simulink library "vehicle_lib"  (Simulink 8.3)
settings: Solver=ode45  StartTime=0.0  StopTime=10.0  RelTol=1e-3
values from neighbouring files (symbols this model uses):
  ambient = class_REVS_ambient    [ambient_param.m]    (also in REVS_run_preproc.m)
  brake = struct(	'max_torque_Nm',[], 						'proportion_norm',1.0, 						'inertia_kgm2',0.0)    [class_REVS_drive_axle.m]
  driver = class_REVS_driver    [driver_param.m]    (also in REVS_run_preproc.m)
  final_drive = struct(	'gear_ratio',[], 								'efficiency_norm',[], 								'inertia_kgm2',[] )    [class_REVS_drive_axle.m]
  tire = struct(	'radius_m',[], 						'rolling_resistance_coefficient',0, 						'vehicle_weight_norm',1.0,  						'wheel_slip_torque_Nm',[],  						'inertia_kgm2',0.0)    [class_REVS_drive_axle.m]
  vehicle = class_REVS_vehicle    [vehicle_standard_car.m]
  vehicle_use_abc_roadload = true    [vehicle_standard_car.m]
undefined symbols (not defined in the file or in its folder): REVS, shaft
libraries: vehicle_lib x24, general_lib x13, audit_lib x12, simulink x7

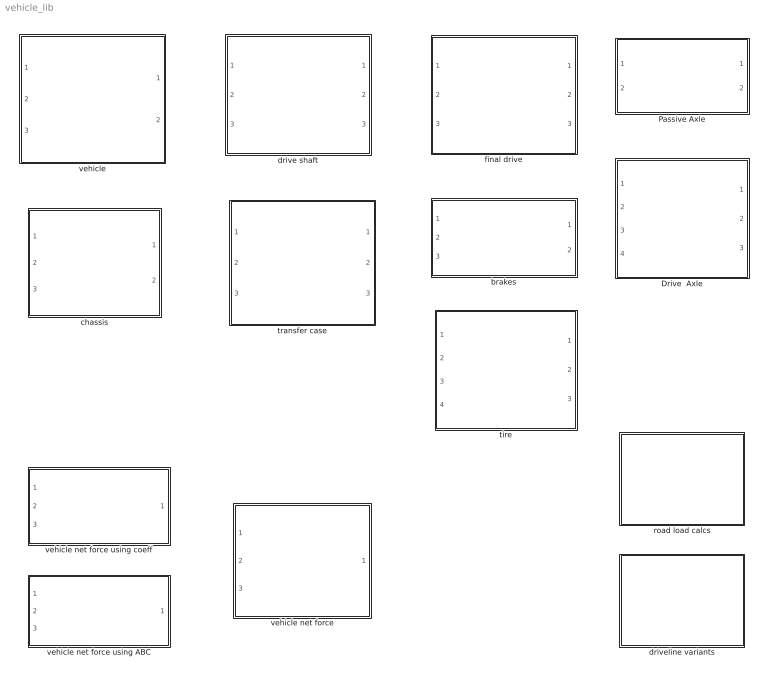
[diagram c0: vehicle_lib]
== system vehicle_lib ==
  Drive  Axle : Subsystem
  Passive Axle : Subsystem
  brakes : Subsystem
  chassis : Subsystem
  drive shaft : Subsystem
  driveline variants : Subsystem
  final drive : Subsystem
  road load calcs : Subsystem
  tire : Subsystem
  transfer case : Subsystem
  vehicle : Subsystem
  vehicle net force : Subsystem  Variant=on
  vehicle net force using ABC : Subsystem  VariantControl=vehicle_use_abc_roadload == true
  vehicle net force using coeff : Subsystem

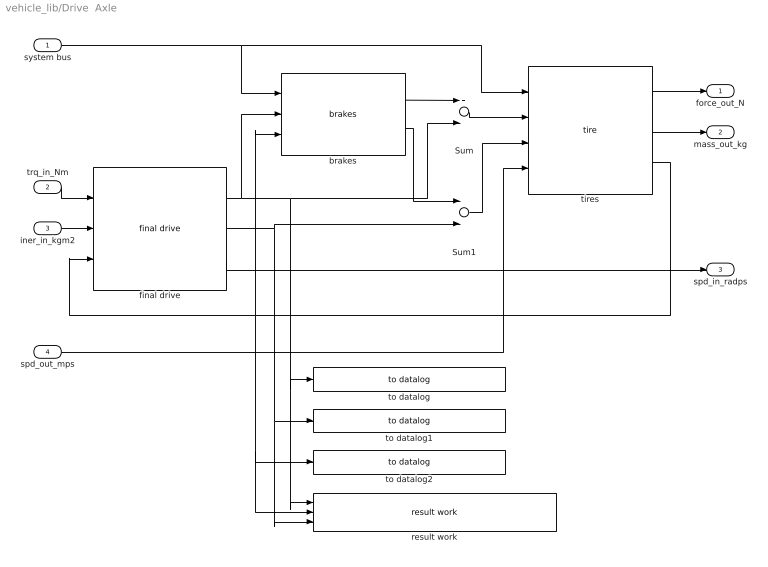
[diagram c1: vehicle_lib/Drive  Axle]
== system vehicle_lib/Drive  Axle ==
  system bus : Inport
  trq_in_Nm : Inport  Port=2
  iner_in_kgm2 : Inport  Port=3
  spd_out_mps : Inport  Port=4
  Sum : Sum
  Sum1 : Sum
  brakes : vehicle_lib/brakes  base_name=drive_axle1__brake  brake=axle.brake
  final drive : vehicle_lib/final drive  base_name=drive_axle1__final_drive  final_drive=axle.final_drive
  result work : general_lib/result work  ResultSignalName=axle_output_pos_work_kJ
  tires : vehicle_lib/tire  base_name=drive_axle1__tire  tire=axle.tire
  to datalog : general_lib/to datalog  VarName=final_drive.output_torque_Nm  WorkspaceName=datalog__final_drive__output_torque_Nm  VerboseLevel=0  VerboseSignal=REVS.verbose
  to datalog1 : general_lib/to datalog  VarName=final_drive.output_inertia_kgm2  WorkspaceName=datalog__final_drive__output_inertia_kgm2  VerboseLevel=0  VerboseSignal=REVS.verbose
  to datalog2 : general_lib/to datalog  VarName=final_drive.output_speed_radps  WorkspaceName=datalog__final_drive__output_speed_radps  VerboseLevel=0  VerboseSignal=REVS.verbose
  force_out_N : Outport
  mass_out_kg : Outport  Port=2
  spd_in_radps : Outport  Port=3
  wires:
  tires/2 -> mass_out_kg/1
  tires/1 -> force_out_N/1
  tires/3 -> result work/2, to datalog2/1, final drive/3, brakes/3
  spd_out_mps/1 -> tires/4
  system bus/1 -> tires/1, brakes/1
  Sum/1 -> tires/2
  brakes/1 -> Sum/1
  Sum1/1 -> tires/3
  brakes/2 -> Sum1/1
  trq_in_Nm/1 -> final drive/1
  iner_in_kgm2/1 -> final drive/2
  final drive/1 -> result work/1, to datalog/1, Sum/2, brakes/2
  final drive/2 -> result work/3, to datalog1/1, Sum1/2
  final drive/3 -> spd_in_radps/1

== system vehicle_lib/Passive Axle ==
  system bus : Inport
  spd_out_mps : Inport  Port=2
  Constant : Constant  Value=0
  brakes : vehicle_lib/brakes  base_name=steer_axle__brake  brake=axle.brake
  tires : vehicle_lib/tire  base_name=steer_axle__tire  tire=axle.tire
  force_out_N : Outport
  mass_out_kg : Outport  Port=2
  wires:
  brakes/1 -> tires/2
  system bus/1 -> tires/1, brakes/1
  brakes/2 -> tires/3
  spd_out_mps/1 -> tires/4
  tires/3 -> brakes/3
  tires/1 -> force_out_N/1
  tires/2 -> mass_out_kg/1
  Constant/1 -> brakes/2

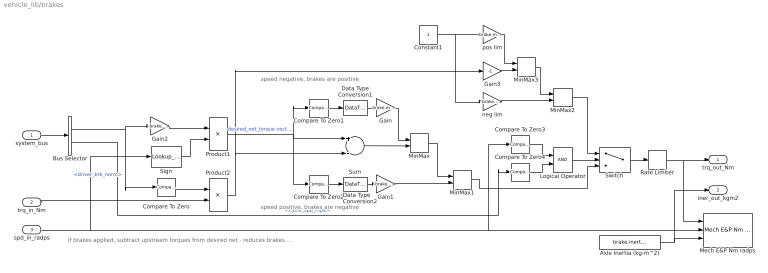
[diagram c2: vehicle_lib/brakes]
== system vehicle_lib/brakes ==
  note: speed negative, brakes are positive
  note: speed positive, brakes are negative
  note: if brakes applied, subtract upstream torques from desired net - reduces brakes for regen, increases if positive torques
  system_bus : Inport
  trq_in_Nm : Inport  Port=2
  spd_in_radps : Inport  Port=3
  Axle Inertia (kg-m^2) : Constant  Value=brake.inertia_kgm2
  Bus Selector : BusSelector  OutputSignals=driver.driver_brk_norm,driver.cycle_spd_mps
  Compare To Zero3 : simulink/Logic and Bit Operations/Compare To Zero  relop===  OutDataTypeStr=boolean
  Compare To Zero4 : simulink/Logic and Bit Operations/Compare To Zero  relop=<=  OutDataTypeStr=boolean
  Compare To Zero : simulink/Logic and Bit Operations/Compare To Zero  relop=>  OutDataTypeStr=boolean
  Compare To Zero1 : simulink/Logic and Bit Operations/Compare To Zero  relop=>  OutDataTypeStr=boolean
  Compare To Zero2 : simulink/Logic and Bit Operations/Compare To Zero  relop=<  OutDataTypeStr=boolean
  Constant1 : Constant
  Data Type Conversion1 : DataTypeConversion
  Data Type Conversion2 : DataTypeConversion
  Gain : Gain  Gain=brake.max_torque_Nm
  Gain1 : Gain  Gain=-brake.max_torque_Nm
  Gain2 : Gain  Gain=-brake.max_torque_Nm
  Gain3 : Gain  Gain=-1
  Logical Operator : Logic  AllPortsSameDT=off  OutDataTypeStr=boolean
  Mech E&P Nm radps : audit_lib/Mech E&P Nm radps  base_name=drive_axle1__brake  VerboseSignal=REVS.verbose
  MinMax : MinMax  Inputs=2  ZeroCross=off
  MinMax1 : MinMax  Function=max  Inputs=2  ZeroCross=off
  MinMax2 : MinMax  Function=max  Inputs=2  ZeroCross=off
  MinMax3 : MinMax  Inputs=2  ZeroCross=off
  Product1 : Product
  Product2 : Product
  Rate Limiter : RateLimiter  RisingSlewLimit=brake.max_torque_Nm  FallingSlewLimit=-brake.max_torque_Nm  SampleTimeMode=inherited
  Sign : Lookup_n-D  NumberOfTableDimensions=1  BreakpointsForDimension1=[-eps 0 eps]  BeginIndexSearchUsingPreviousIndexResult=on  Table=[-1 1 1]  ExtrapMethod=Clip  UseLastTableValue=on  RndMeth=Simplest
  Sum : Sum  Inputs=+-
  Switch : Switch  Criteria=u2 > Threshold
  neg lim : Gain  Gain=-brake.max_torque_Nm
  pos lim : Gain  Gain=brake.max_torque_Nm
  trq_out_Nm : Outport
  iner_out_kgm2 : Outport  Port=2
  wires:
  Constant1/1 -> pos lim/1, neg lim/1
  Switch/1 -> Rate Limiter/1
  MinMax2/1 -> Switch/1
  MinMax3/1 -> MinMax2/1
  neg lim/1 -> MinMax2/2
  Gain3/1 -> MinMax3/2
  pos lim/1 -> MinMax3/1
  MinMax1/1 -> Switch/3
  Logical Operator/1 -> Switch/2
  Product1/1 -> Compare To Zero2/1, Sum/1, Compare To Zero1/1  "desired_net_torque vector"
  Bus Selector/2 -> Compare To Zero4/1  "<cycle_spd_mps>"
  Compare To Zero4/1 -> Logical Operator/2
  Compare To Zero3/1 -> Logical Operator/1
  Rate Limiter/1 -> Mech E&P Nm radps/1, trq_out_Nm/1
  MinMax/1 -> MinMax1/1
  Gain2/1 -> Product1/1
  Sign/1 -> Product1/2
  system_bus/1 -> Bus Selector/1
  Axle Inertia (kg-m^2)/1 -> iner_out_kgm2/1, Mech E&P Nm radps/3
  spd_in_radps/1 -> Mech E&P Nm radps/2, Compare To Zero3/1, Sign/1
  Bus Selector/1 -> Compare To Zero/1, Gain2/1  "<driver_brk_norm>"
  trq_in_Nm/1 -> Product2/2
  Compare To Zero/1 -> Product2/1
  Product2/1 -> Sum/2, Gain3/1
  Sum/1 -> MinMax/2
  Compare To Zero1/1 -> Data Type Conversion1/1
  Gain/1 -> MinMax/1
  Compare To Zero2/1 -> Data Type Conversion2/1
  Gain1/1 -> MinMax1/2
  Data Type Conversion1/1 -> Gain/1
  Data Type Conversion2/1 -> Gain1/1

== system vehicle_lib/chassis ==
  system_bus : Inport
  force_in_N : Inport  Port=2
  mass_in_kg : Inport  Port=3
  Bus Creator : BusCreator  Inputs=2
  vehicle net force : vehicle_lib/vehicle net force
  vehicle speed integrator : Subsystem
  bus_out : Outport
  veh_spd_mps : Outport  Port=2
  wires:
  vehicle speed integrator/2(veh_dist_m) -> Bus Creator/2  "veh_dist_m"
  vehicle speed integrator/1(veh_spd_mps) -> veh_spd_mps/1, vehicle net force/3, Bus Creator/1  "veh_spd_mps"
  vehicle net force/1 -> vehicle speed integrator/1(force_out_N)
  mass_in_kg/1 -> vehicle speed integrator/2(mass_in_kg)
  force_in_N/1 -> vehicle net force/2
  system_bus/1 -> vehicle net force/1
  Bus Creator/1 -> bus_out/1  "vehicle"

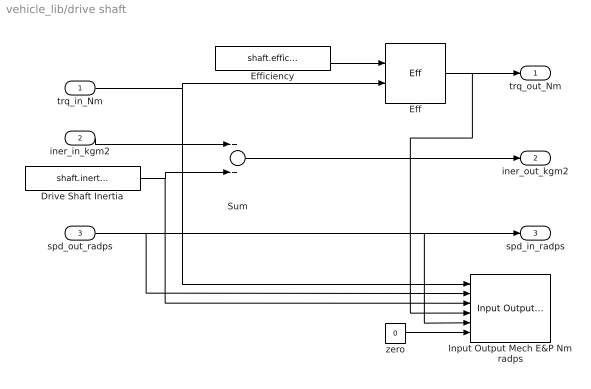
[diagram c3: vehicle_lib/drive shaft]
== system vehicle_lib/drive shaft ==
  trq_in_Nm : Inport
  iner_in_kgm2 : Inport  Port=2
  spd_out_radps : Inport  Port=3
  Drive Shaft Inertia : Constant  Value=shaft.inertia_kgm2
  Eff : general_lib/Eff
  Efficiency : Constant  Value=shaft.efficiency_norm
  Input Output Mech E&P Nm radps : audit_lib/Input Output Mech E&P Nm radps  base_name=driveshaft  VerboseSignal=REVS.verbose
  Sum : Sum
  zero : Constant  Value=0
  trq_out_Nm : Outport
  iner_out_kgm2 : Outport  Port=2
  spd_in_radps : Outport  Port=3
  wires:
  iner_in_kgm2/1 -> Sum/1
  Sum/1 -> iner_out_kgm2/1
  Drive Shaft Inertia/1 -> Input Output Mech E&P Nm radps/3, Sum/2
  spd_out_radps/1 -> Input Output Mech E&P Nm radps/2, Input Output Mech E&P Nm radps/5, spd_in_radps/1
  trq_in_Nm/1 -> Eff/2, Input Output Mech E&P Nm radps/1
  Efficiency/1 -> Eff/1
  Eff/1 -> Input Output Mech E&P Nm radps/4, trq_out_Nm/1
  zero/1 -> Input Output Mech E&P Nm radps/6

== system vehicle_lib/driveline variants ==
  driveline : Subsystem  Variant=on
  one axle drive : Subsystem  VariantControl=vehicle_driveline_type == enum_driveline_type.one_axle_drive

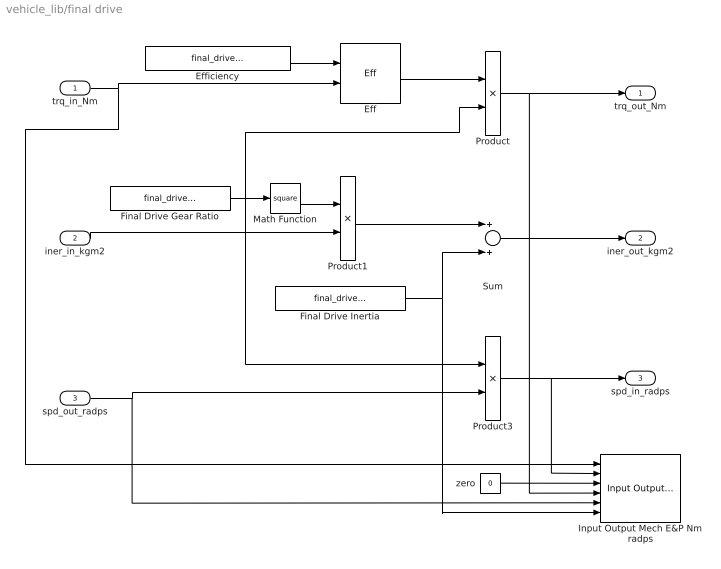
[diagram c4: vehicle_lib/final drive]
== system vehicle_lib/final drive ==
  trq_in_Nm : Inport
  iner_in_kgm2 : Inport  Port=2
  spd_out_radps : Inport  Port=3
  Eff : general_lib/Eff
  Efficiency : Constant  Value=final_drive.efficiency_norm
  Final Drive Gear Ratio : Constant  Value=final_drive.gear_ratio
  Final Drive Inertia : Constant  Value=final_drive.inertia_kgm2
  Input Output Mech E&P Nm radps : audit_lib/Input Output Mech E&P Nm radps  base_name=device  VerboseSignal=REVS.verbose
  Math Function : Math  Operator=square
  Product : Product
  Product1 : Product
  Product3 : Product
  Sum : Sum
  zero : Constant  Value=0
  trq_out_Nm : Outport
  iner_out_kgm2 : Outport  Port=2
  spd_in_radps : Outport  Port=3
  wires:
  Sum/1 -> iner_out_kgm2/1
  Product/1 -> Input Output Mech E&P Nm radps/4, trq_out_Nm/1
  Final Drive Inertia/1 -> Input Output Mech E&P Nm radps/6, Sum/2
  Product1/1 -> Sum/1
  iner_in_kgm2/1 -> Product1/2
  trq_in_Nm/1 -> Eff/2, Input Output Mech E&P Nm radps/1
  Final Drive Gear Ratio/1 -> Product/2, Math Function/1, Product3/1
  Math Function/1 -> Product1/1
  spd_out_radps/1 -> Input Output Mech E&P Nm radps/5, Product3/2
  Product3/1 -> Input Output Mech E&P Nm radps/2, spd_in_radps/1
  Efficiency/1 -> Eff/1
  Eff/1 -> Product/1
  zero/1 -> Input Output Mech E&P Nm radps/3

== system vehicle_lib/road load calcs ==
  acceleration force : Subsystem
  aerodynamic drag : Subsystem
  driver road load by ABC : Subsystem  InitFcn=if GEM_verbose disp('Using driver roadload by coastdown...'); end  VariantControl=variants_driver_roadload_ABC
  driver road load by Cd-Crr : Subsystem  InitFcn=if GEM_verbose disp('Using driver roadload by coefficients...'); end  VariantControl=variants_driver_roadload_coeff
  gradient force : Subsystem
  road load by ABC : Subsystem
  rolling resistance : Subsystem

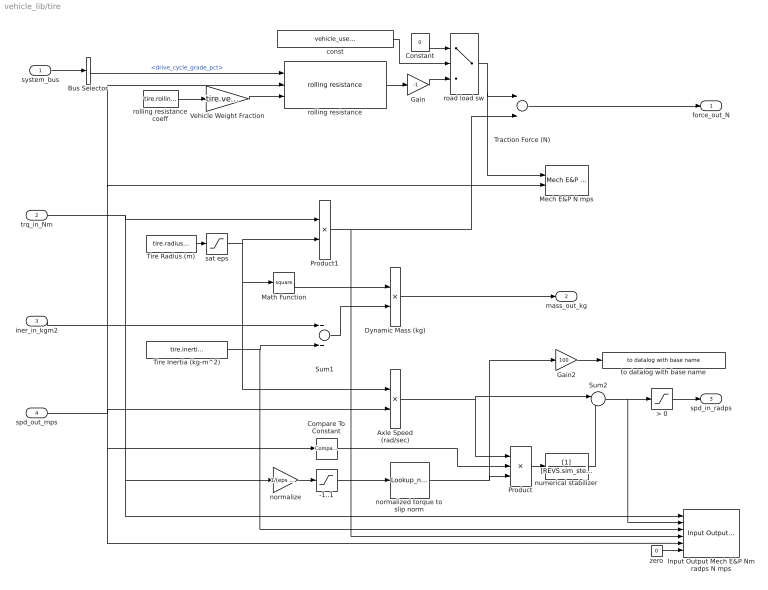
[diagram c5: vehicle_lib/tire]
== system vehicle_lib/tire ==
  system_bus : Inport
  trq_in_Nm : Inport  Port=2
  iner_in_kgm2 : Inport  Port=3
  spd_out_mps : Inport  Port=4
  -1..1 : Saturate  UpperLimit=1  LowerLimit=-1  ZeroCross=off
  > 0 : Saturate  UpperLimit=Inf  LowerLimit=0  ZeroCross=off
  Axle Speed (rad/sec) : Product  Inputs=/*
  Bus Selector : BusSelector  OutputSignals=ambient.drive_cycle_grade_pct
  Compare To Constant : simulink/Logic and Bit Operations/Compare To Constant  relop=>=  const=0.1  OutDataTypeStr=boolean
  Constant : Constant  Value=0
  Dynamic Mass (kg) : Product  Inputs=/*
  Gain : Gain  Gain=-1
  Gain2 : Gain  Gain=100
  Input Output Mech E&P Nm radps N mps : audit_lib/Input Output Mech E&P Nm radps N mps  base_name=drive_axle1__tire  VerboseSignal=REVS.verbose
  Math Function : Math  Operator=square
  Mech E&P N mps : audit_lib/Mech E&P N mps0  base_name=drive_axle1__tire__rolling_drag  VerboseSignal=REVS.verbose
  Product : Product  Inputs=3
  Product1 : Product  Inputs=*/
  Sum1 : Sum
  Sum2 : Sum  Inputs=|++
  Tire Inertia (kg-m^2) : Constant  Value=tire.inertia_kgm2
  Tire Radius (m) : Constant  Value=tire.radius_m
  Traction Force (N) : Sum
  Vehicle Weight Fraction : Gain  Gain=tire.vehicle_weight_norm
  const : Constant  Value=vehicle_use_abc_roadload
  normalize : Gain  Gain=1/(eps + tire.wheel_slip_torque_Nm)
  normalized torque to slip norm : Lookup_n-D  NumberOfTableDimensions=1  BreakpointsForDimension1=[-0.999866216844745 -0.99978414282011 -0.99807408909811 -0.994136683198638 -0.987125284420945 -0.975823606608682 -0.958455233159564 -0.932389621966496 -0.893705646328621 -0.836611821621369 -0.752906045607232 -0.632208437687154 -0.464747309940849 -0.248771439727253 0 0.248771439727253 0.464747309940849 0.632208437687154 0.752906045607232 0.836611821621369 0.893705646328621 0.932389621966496 0.95845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  IndexSearchMethod=Linear search  BeginIndexSearchUsingPreviousIndexResult=on  Table=-0.14 : 0.01 : 0.14  ExtrapMethod=Clip  UseLastTableValue=on  RndMeth=Simplest
  numerical stabilizer : TransferFcn  Denominator=[REVS.sim_step_time_secs 1]
  road load sw : Switch  Criteria=u2 > Threshold  ZeroCross=off
  rolling resistance : vehicle_lib/road load calcs/rolling resistance
  rolling resistance coeff : Constant  Value=tire.rolling_resistance_coefficient
  sat eps : Saturate  UpperLimit=Inf  LowerLimit=eps  ZeroCross=off
  to datalog with base name : general_lib/to datalog with base name  varName=slip_pct  baseName=base_name  VerboseLevel=1  VerboseSignal=REVS.verbose
  zero : Constant  Value=0
  force_out_N : Outport
  mass_out_kg : Outport  Port=2
  spd_in_radps : Outport  Port=3
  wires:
  normalized torque to slip norm/1 -> Product/3, Gain2/1
  -1..1/1 -> normalized torque to slip norm/1
  Compare To Constant/1 -> Product/2
  normalize/1 -> -1..1/1
  Gain2/1 -> to datalog with base name/1
  > 0/1 -> spd_in_radps/1
  spd_out_mps/1 -> Mech E&P N mps/2, rolling resistance/2, Axle Speed (rad/sec)/2, Input Output Mech E&P Nm radps N mps/5, Compare To Constant/1
  numerical stabilizer/1 -> Sum2/2
  Sum2/1 -> > 0/1, Input Output Mech E&P Nm radps N mps/2
  Product/1 -> numerical stabilizer/1
  Traction Force (N)/1 -> force_out_N/1
  trq_in_Nm/1 -> Product1/1, normalize/1, Input Output Mech E&P Nm radps N mps/1
  Axle Speed (rad/sec)/1 -> Product/1, Sum2/1
  Vehicle Weight Fraction/1 -> rolling resistance/3
  rolling resistance/1 -> Gain/1
  Bus Selector/1 -> rolling resistance/1  "<drive_cycle_grade_pct>"
  rolling resistance coeff/1 -> Vehicle Weight Fraction/1
  Dynamic Mass (kg)/1 -> mass_out_kg/1
  Sum1/1 -> Dynamic Mass (kg)/2
  Tire Inertia (kg-m^2)/1 -> Sum1/2, Input Output Mech E&P Nm radps N mps/3
  iner_in_kgm2/1 -> Sum1/1
  Tire Radius (m)/1 -> sat eps/1
  system_bus/1 -> Bus Selector/1
  Product1/1 -> Input Output Mech E&P Nm radps N mps/4, Traction Force (N)/2
  road load sw/1 -> Mech E&P N mps/1, Traction Force (N)/1
  Gain/1 -> road load sw/3
  const/1 -> road load sw/2
  Constant/1 -> road load sw/1
  sat eps/1 -> Axle Speed (rad/sec)/1, Math Function/1, Product1/2
  Math Function/1 -> Dynamic Mass (kg)/1
  zero/1 -> Input Output Mech E&P Nm radps N mps/6

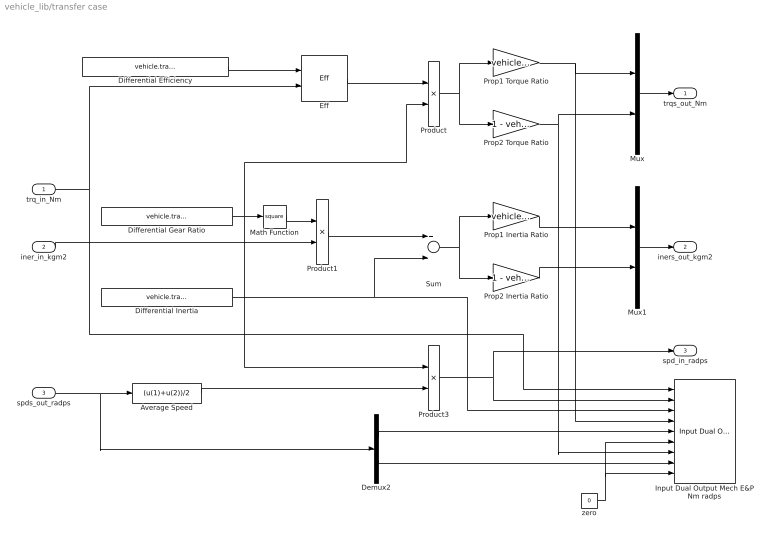
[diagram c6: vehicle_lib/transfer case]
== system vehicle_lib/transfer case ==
  trq_in_Nm : Inport
  iner_in_kgm2 : Inport  Port=2
  spds_out_radps : Inport  Port=3
  Average Speed : Fcn  Expr=(u(1)+u(2))/2
  Demux2 : Demux  Outputs=2
  Differential Efficiency : Constant  Value=vehicle.transfer_case.efficiency_norm
  Differential Gear Ratio : Constant  Value=vehicle.transfer_case.gear_ratio
  Differential Inertia : Constant  Value=vehicle.transfer_case.inertia_kgm2
  Eff : general_lib/Eff
  Input Dual Output Mech E&P Nm radps : audit_lib/Input Dual Output Mech E&P Nm radps  base_name=transfer_case  VerboseSignal=REVS.verbose
  Math Function : Math  Operator=square
  Mux : Mux  Inputs=2
  Mux1 : Mux  Inputs=2
  Product : Product
  Product1 : Product
  Product3 : Product
  Prop1 Inertia Ratio : Gain  Gain=vehicle.transfer_case.prop1_torque_ratio
  Prop1 Torque Ratio : Gain  Gain=vehicle.transfer_case.prop1_torque_ratio
  Prop2 Inertia Ratio : Gain  Gain=1 - vehicle.transfer_case.prop1_torque_ratio
  Prop2 Torque Ratio : Gain  Gain=1 - vehicle.transfer_case.prop1_torque_ratio
  Sum : Sum
  zero : Constant  Value=0
  trqs_out_Nm : Outport
  iners_out_kgm2 : Outport  Port=2
  spd_in_radps : Outport  Port=3
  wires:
  Demux2/2 -> Input Dual Output Mech E&P Nm radps/8
  Demux2/1 -> Input Dual Output Mech E&P Nm radps/5
  Average Speed/1 -> Product3/2
  spds_out_radps/1 -> Average Speed/1, Demux2/1
  Math Function/1 -> Product1/1
  Differential Gear Ratio/1 -> Math Function/1, Product/2, Product3/1
  trq_in_Nm/1 -> Eff/2, Input Dual Output Mech E&P Nm radps/1
  Eff/1 -> Product/1
  iner_in_kgm2/1 -> Product1/2
  Product1/1 -> Sum/1
  Differential Inertia/1 -> Sum/2, Input Dual Output Mech E&P Nm radps/3
  Product3/1 -> Input Dual Output Mech E&P Nm radps/2, spd_in_radps/1
  Product/1 -> Prop1 Torque Ratio/1, Prop2 Torque Ratio/1
  Sum/1 -> Prop1 Inertia Ratio/1, Prop2 Inertia Ratio/1
  Prop1 Torque Ratio/1 -> Input Dual Output Mech E&P Nm radps/4, Mux/1
  Prop2 Torque Ratio/1 -> Input Dual Output Mech E&P Nm radps/7, Mux/2
  Prop1 Inertia Ratio/1 -> Mux1/1
  Prop2 Inertia Ratio/1 -> Mux1/2
  Mux/1 -> trqs_out_Nm/1
  Mux1/1 -> iners_out_kgm2/1
  Differential Efficiency/1 -> Eff/1
  zero/1 -> Input Dual Output Mech E&P Nm radps/6, Input Dual Output Mech E&P Nm radps/9

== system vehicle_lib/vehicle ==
  system_bus : Inport
  trq_in_Nm : Inport  Port=2
  iner_in_kgm2 : Inport  Port=3
  Bus Creator1 : BusCreator  Inputs=1
  chassis : vehicle_lib/chassis  SystemSampleTime=-1
  driveline : vehicle_lib/driveline variants/driveline
  bus_out : Outport
  spd_in_radps : Outport  Port=2
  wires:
  chassis/2 -> driveline/4
  system_bus/1 -> driveline/1, chassis/1
  trq_in_Nm/1 -> driveline/2
  iner_in_kgm2/1 -> driveline/3
  driveline/3 -> spd_in_radps/1
  driveline/1 -> chassis/2
  driveline/2 -> chassis/3
  chassis/1 -> Bus Creator1/1  "chassis"
  Bus Creator1/1 -> bus_out/1  "vehicle"

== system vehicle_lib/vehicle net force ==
  note: 1) Only subsystems can be added as variant choices at this level 2) Blocks cannot be connected at this level as connectivity is automatically determined at simulation, based on the active variant
  system_bus : Inport
  force_in_N : Inport  Port=2
  chs_spd_mps : Inport  Port=3
  vehicle net force using ABC : vehicle_lib/vehicle net force using ABC  VariantControl=vehicle_use_abc_roadload == true
  vehicle net force using coeff : vehicle_lib/vehicle net force using coeff  VariantControl=vehicle_use_abc_roadload == false
  force_out_N : Outport

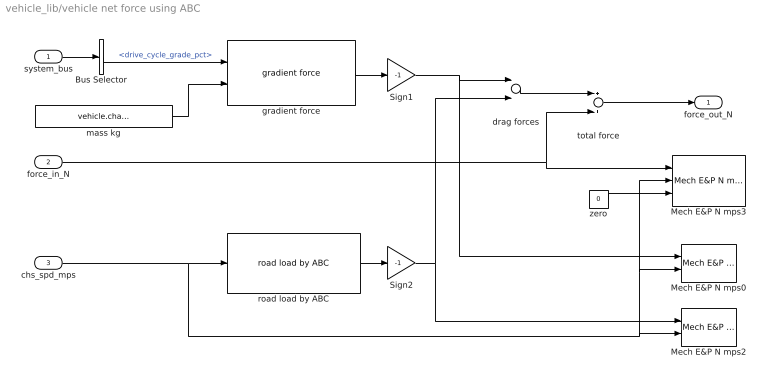
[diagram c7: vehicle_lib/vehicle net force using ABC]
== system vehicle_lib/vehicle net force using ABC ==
  system_bus : Inport
  force_in_N : Inport  Port=2
  chs_spd_mps : Inport  Port=3
  Bus Selector : BusSelector  OutputSignals=ambient.drive_cycle_grade_pct
  Mech E&P N mps0 : audit_lib/Mech E&P N mps0  base_name=vehicle.gradient_drag  VerboseSignal=REVS.verbose
  Mech E&P N mps2 : audit_lib/Mech E&P N mps0  base_name=vehicle.ABC_drag  VerboseSignal=REVS.verbose
  Mech E&P N mps3 : audit_lib/Mech E&P N mps  base_name=vehicle.input  VerboseSignal=REVS.verbose
  Sign1 : Gain  Gain=-1
  Sign2 : Gain  Gain=-1
  drag forces : Sum
  gradient force : vehicle_lib/road load calcs/gradient force
  mass kg : Constant  Value=vehicle.chassis.mass_static_kg
  road load by ABC : vehicle_lib/road load calcs/road load by ABC
  total force : Sum
  zero : Constant  Value=0
  force_out_N : Outport
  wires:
  zero/1 -> Mech E&P N mps3/3
  chs_spd_mps/1 -> road load by ABC/1, Mech E&P N mps2/2, Mech E&P N mps0/2, Mech E&P N mps3/2
  gradient force/1 -> Sign1/1
  drag forces/1 -> total force/1
  Sign1/1 -> Mech E&P N mps0/1, drag forces/1
  Bus Selector/1 -> gradient force/1  "<drive_cycle_grade_pct>"
  system_bus/1 -> Bus Selector/1
  mass kg/1 -> gradient force/2
  force_in_N/1 -> total force/2, Mech E&P N mps3/1
  total force/1 -> force_out_N/1
  road load by ABC/1 -> Sign2/1
  Sign2/1 -> drag forces/2, Mech E&P N mps2/1

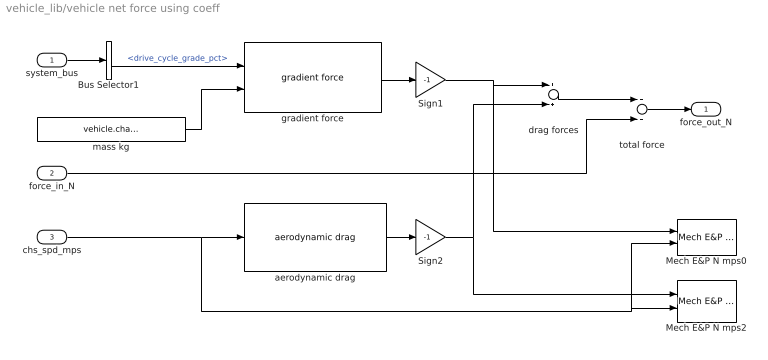
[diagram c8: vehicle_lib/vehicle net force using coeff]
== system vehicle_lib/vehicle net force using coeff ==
  system_bus : Inport
  force_in_N : Inport  Port=2
  chs_spd_mps : Inport  Port=3
  Bus Selector1 : BusSelector  OutputSignals=ambient.drive_cycle_grade_pct
  Mech E&P N mps0 : audit_lib/Mech E&P N mps0  base_name=vehicle.gradient_drag  VerboseSignal=REVS.verbose
  Mech E&P N mps2 : audit_lib/Mech E&P N mps0  base_name=vehicle.aerodynamic_drag  VerboseSignal=REVS.verbose
  Sign1 : Gain  Gain=-1
  Sign2 : Gain  Gain=-1
  aerodynamic drag : vehicle_lib/road load calcs/aerodynamic drag
  drag forces : Sum
  gradient force : vehicle_lib/road load calcs/gradient force
  mass kg : Constant  Value=vehicle.chassis.mass_static_kg
  total force : Sum
  force_out_N : Outport
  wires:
  total force/1 -> force_out_N/1
  force_in_N/1 -> total force/2
  mass kg/1 -> gradient force/2
  system_bus/1 -> Bus Selector1/1
  Bus Selector1/1 -> gradient force/1  "<drive_cycle_grade_pct>"
  Sign1/1 -> drag forces/1, Mech E&P N mps0/1
  drag forces/1 -> total force/1
  gradient force/1 -> Sign1/1
  aerodynamic drag/1 -> Sign2/1
  Sign2/1 -> Mech E&P N mps2/1, drag forces/2
  chs_spd_mps/1 -> aerodynamic drag/1, Mech E&P N mps0/2, Mech E&P N mps2/2

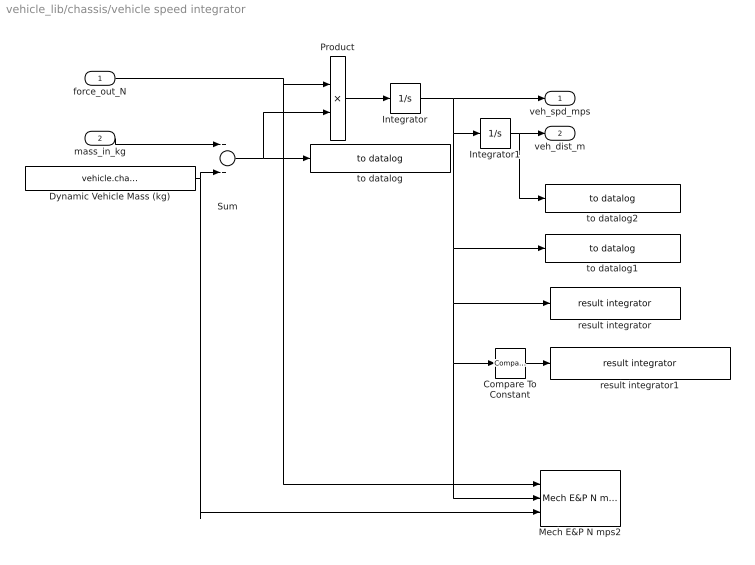
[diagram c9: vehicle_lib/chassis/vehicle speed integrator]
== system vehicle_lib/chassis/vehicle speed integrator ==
  force_out_N : Inport
  mass_in_kg : Inport  Port=2
  Compare To Constant : simulink/Logic and Bit Operations/Compare To Constant  relop=<=  const=0.1  OutDataTypeStr=boolean
  Dynamic Vehicle Mass (kg) : Constant  Value=vehicle.chassis.mass_dynamic_kg
  Integrator : Integrator  LimitOutput=on  UpperSaturationLimit=Inf  LowerSaturationLimit=0
  Integrator1 : Integrator  LimitOutput=on  UpperSaturationLimit=Inf  LowerSaturationLimit=0  ZeroCross=off
  Mech E&P N mps2 : audit_lib/Mech E&P N mps  base_name=vehicle.output  VerboseSignal=REVS.verbose
  Product : Product  Inputs=*/
  Sum : Sum  Inputs=2
  result integrator : general_lib/result integrator  ResultSignalName=distance_m
  result integrator1 : general_lib/result integrator  ResultSignalName=stopped_time_secs
  to datalog : general_lib/to datalog  VarName=vehicle__dynamic_mass_kg  WorkspaceName=datalog__vehicle__dynamic_mass_kg  VerboseLevel=1  VerboseSignal=REVS.verbose
  to datalog1 : general_lib/to datalog  VarName=vehicle__speed_mps  WorkspaceName=datalog__vehicle__speed_mps  VerboseLevel=0  VerboseSignal=REVS.verbose
  to datalog2 : general_lib/to datalog  VarName=vehicle__distance_m  WorkspaceName=datalog__vehicle__distance_m  VerboseLevel=0  VerboseSignal=REVS.verbose
  veh_spd_mps : Outport
  veh_dist_m : Outport  Port=2
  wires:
  force_out_N/1 -> Product/1, Mech E&P N mps2/1
  Product/1 -> Integrator/1
  Integrator/1 -> to datalog1/1, Mech E&P N mps2/2, Compare To Constant/1, result integrator/1, Integrator1/1, veh_spd_mps/1
  Dynamic Vehicle Mass (kg)/1 -> Sum/2, Mech E&P N mps2/3
  mass_in_kg/1 -> Sum/1
  Sum/1 -> to datalog/1, Product/2
  Integrator1/1 -> to datalog2/1, veh_dist_m/1
  Compare To Constant/1 -> result integrator1/1

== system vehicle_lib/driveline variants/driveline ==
  note: 1) Only subsystems can be added as variant choices at this level 2) Blocks cannot be connected at this level as connectivity is automatically determined at simulation, based on the active variant
  system_bus : Inport
  trq_in_Nm : Inport  Port=2
  iner_in_kgm2 : Inport  Port=3
  spd_out_mps : Inport  Port=4
  one axle drive : vehicle_lib/driveline variants/one axle drive  VariantControl=vehicle_driveline_type == enum_driveline_type.one_axle_drive
  force_out_N : Outport
  mass_out_kg : Outport  Port=2
  spd_in_radps : Outport  Port=3

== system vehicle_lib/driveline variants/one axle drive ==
  system_bus : Inport
  trq_in_Nm : Inport  Port=2
  iner_in_kgm2 : Inport  Port=3
  spd_out_mps : Inport  Port=4
  Drive  Axle : vehicle_lib/Drive  Axle  base_name=drive_axle1  axle=vehicle.drive_axle1
  force_out_N : Outport
  mass_out_kg : Outport  Port=2
  spd_in_radps : Outport  Port=3
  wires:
  Drive  Axle/1 -> force_out_N/1
  Drive  Axle/2 -> mass_out_kg/1
  Drive  Axle/3 -> spd_in_radps/1
  system_bus/1 -> Drive  Axle/1
  trq_in_Nm/1 -> Drive  Axle/2
  iner_in_kgm2/1 -> Drive  Axle/3
  spd_out_mps/1 -> Drive  Axle/4

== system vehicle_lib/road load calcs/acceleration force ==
  veh_spd_mps : Inport
  mass_kg : Inport  Port=2
  Acceleration 1 : Derivative
  Acceleration Force (N)1 : Product
  low pass filter : TransferFcn  Denominator=[driver.pedal_response 1]
  sat >= 0 : Saturate  UpperLimit=Inf  LowerLimit=0
  accel_force_N : Outport
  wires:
  low pass filter/1 -> Acceleration Force (N)1/2
  mass_kg/1 -> low pass filter/1
  Acceleration 1/1 -> sat >= 0/1
  veh_spd_mps/1 -> Acceleration 1/1
  Acceleration Force (N)1/1 -> accel_force_N/1
  sat >= 0/1 -> Acceleration Force (N)1/1

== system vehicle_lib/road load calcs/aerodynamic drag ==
  veh_spd_mps : Inport
  Aero Drag Force (N) : Product  Inputs=5
  Air Density (kg/m^3) : Constant  Value=ambient.air_density_kgpm3
  Drag Coefficient : Constant  Value=vehicle.chassis.aerodynamic_drag_coeff
  Frontal Area (m^2) : Constant  Value=vehicle.chassis.frontal_area_m2
  Gain : Gain  Gain=0.5
  Math Function : Math  Operator=square
  Sign : Signum  ZeroCross=off
  aero_force_N : Outport
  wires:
  Math Function/1 -> Aero Drag Force (N)/1
  Air Density (kg/m^3)/1 -> Aero Drag Force (N)/3
  Frontal Area (m^2)/1 -> Aero Drag Force (N)/4
  Drag Coefficient/1 -> Aero Drag Force (N)/5
  Gain/1 -> Aero Drag Force (N)/2
  Aero Drag Force (N)/1 -> aero_force_N/1
  Sign/1 -> Gain/1
  veh_spd_mps/1 -> Math Function/1, Sign/1

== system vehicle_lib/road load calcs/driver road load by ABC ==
  system_bus : Inport
  veh_spd_des_mps : Inport  Port=2
  Bus Selector : BusSelector  OutputSignals=ambient.driving_grade_pct,vehicle.chassis.veh_dynamic_kg
  Static Vehicle Mass (kg) : Constant  Value=vehicle.chassis.mass_static_kg
  Wheel Radius (m) : Constant  Value=vehicle.tire.prop1_radius_m
  acceleration force : vehicle_lib/road load calcs/acceleration force
  gradient force : vehicle_lib/road load calcs/gradient force
  road load by ABC : vehicle_lib/road load calcs/road load by ABC
  total force demand : Sum  Inputs=+++
  total torque demand : Product
  whl_trq_dmd_road_Nm : Outport
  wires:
  total torque demand/1 -> whl_trq_dmd_road_Nm/1
  acceleration force/1 -> total force demand/3
  Bus Selector/2 -> acceleration force/2  "<veh_dynamic_kg>"
  gradient force/1 -> total force demand/1
  Wheel Radius (m)/1 -> total torque demand/2
  total force demand/1 -> total torque demand/1
  Static Vehicle Mass (kg)/1 -> gradient force/2
  Bus Selector/1 -> gradient force/1  "<driving_grade_pct>"
  system_bus/1 -> Bus Selector/1
  road load by ABC/1 -> total force demand/2
  veh_spd_des_mps/1 -> road load by ABC/1, acceleration force/1

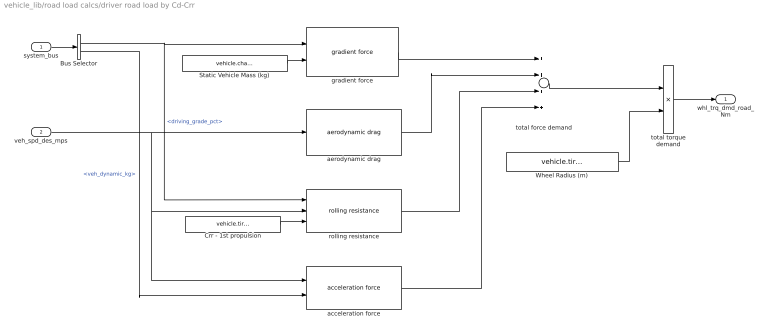
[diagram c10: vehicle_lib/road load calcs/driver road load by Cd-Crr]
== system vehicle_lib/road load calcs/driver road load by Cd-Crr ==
  system_bus : Inport
  veh_spd_des_mps : Inport  Port=2
  Bus Selector : BusSelector  OutputSignals=ambient.driving_grade_pct,vehicle.chassis.veh_dynamic_kg
  Crr - 1st propulsion : Constant  Value=vehicle.tire.prop1_roll_coef
  Static Vehicle Mass (kg) : Constant  Value=vehicle.chassis.mass_static_kg
  Wheel Radius (m) : Constant  Value=vehicle.tire.prop1_radius_m
  acceleration force : vehicle_lib/road load calcs/acceleration force
  aerodynamic drag : vehicle_lib/road load calcs/aerodynamic drag
  gradient force : vehicle_lib/road load calcs/gradient force
  rolling resistance : vehicle_lib/road load calcs/rolling resistance
  total force demand : Sum  Inputs=++++
  total torque demand : Product
  whl_trq_dmd_road_Nm : Outport
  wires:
  veh_spd_des_mps/1 -> aerodynamic drag/1, rolling resistance/2, acceleration force/1
  Bus Selector/2 -> acceleration force/2  "<veh_dynamic_kg>"
  acceleration force/1 -> total force demand/4
  rolling resistance/1 -> total force demand/3
  aerodynamic drag/1 -> total force demand/2
  total torque demand/1 -> whl_trq_dmd_road_Nm/1
  Bus Selector/1 -> gradient force/1, rolling resistance/1  "<driving_grade_pct>"
  system_bus/1 -> Bus Selector/1
  total force demand/1 -> total torque demand/1
  Wheel Radius (m)/1 -> total torque demand/2
  Static Vehicle Mass (kg)/1 -> gradient force/2
  gradient force/1 -> total force demand/1
  Crr - 1st propulsion/1 -> rolling resistance/3

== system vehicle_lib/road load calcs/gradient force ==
  grade_pct : Inport
  mass_kg : Inport  Port=2
  % grade to norm : Gain  Gain=0.01
  Gradient Force (N) : Product  Inputs=3
  Gravitational Acceleration (m/sec^2) : Constant  Value=ambient.gravity_mps2
  Trigonometric Function : Trigonometry  Operator=atan
  Trigonometric Function1 : Trigonometry
  grade_force_N : Outport
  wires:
  grade_pct/1 -> % grade to norm/1
  Trigonometric Function1/1 -> Gradient Force (N)/1
  Gradient Force (N)/1 -> grade_force_N/1
  % grade to norm/1 -> Trigonometric Function/1
  Trigonometric Function/1 -> Trigonometric Function1/1
  Gravitational Acceleration (m/sec^2)/1 -> Gradient Force (N)/2
  mass_kg/1 -> Gradient Force (N)/3

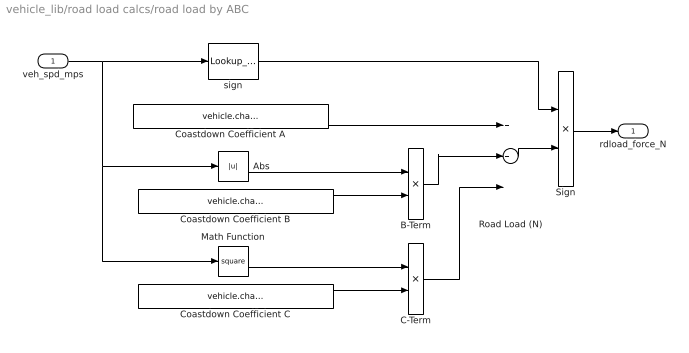
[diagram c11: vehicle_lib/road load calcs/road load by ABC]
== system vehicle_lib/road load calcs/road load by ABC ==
  veh_spd_mps : Inport
  Abs : Abs
  B-Term : Product
  C-Term : Product
  Coastdown Coefficient A : Constant  Value=vehicle.chassis.coastdown_A_N
  Coastdown Coefficient B : Constant  Value=vehicle.chassis.coastdown_B_Npms
  Coastdown Coefficient C : Constant  Value=vehicle.chassis.coastdown_C_Npms2
  Math Function : Math  Operator=square
  Road Load (N) : Sum  Inputs=3
  Sign : Product
  sign : Lookup_n-D  NumberOfTableDimensions=1  BreakpointsForDimension1=[-eps 0 eps]  BeginIndexSearchUsingPreviousIndexResult=on  Table=[-1 1 1]  ExtrapMethod=Clip  UseLastTableValue=on  RndMeth=Simplest
  rdload_force_N : Outport
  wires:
  Road Load (N)/1 -> Sign/2
  Coastdown Coefficient C/1 -> C-Term/2
  B-Term/1 -> Road Load (N)/2
  Sign/1 -> rdload_force_N/1
  C-Term/1 -> Road Load (N)/3
  Coastdown Coefficient B/1 -> B-Term/2
  Coastdown Coefficient A/1 -> Road Load (N)/1
  veh_spd_mps/1 -> sign/1, Math Function/1, Abs/1
  Math Function/1 -> C-Term/1
  Abs/1 -> B-Term/1
  sign/1 -> Sign/1

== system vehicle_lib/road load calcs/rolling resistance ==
  grade_pct : Inport
  veh_spd_mps : Inport  Port=2
  Crr : Inport  Port=3
  % grade to norm : Gain  Gain=0.01
  Gravitational Acceleration (m/sec^2)1 : Constant  Value=ambient.gravity_mps2
  Rolling Resistance Force (N) : Product  Inputs=5
  Sign : Lookup_n-D  NumberOfTableDimensions=1  BreakpointsForDimension1=[-eps 0 eps]  BeginIndexSearchUsingPreviousIndexResult=on  Table=[-1 1 1]  ExtrapMethod=Clip  UseLastTableValue=on  RndMeth=Simplest
  Static Vehicle Mass (kg) : Constant  Value=vehicle.chassis.mass_static_kg
  Trigonometric Function2 : Trigonometry  Operator=atan
  Trigonometric Function3 : Trigonometry  Operator=cos
  " roll_res_force_N" : Outport
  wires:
  grade_pct/1 -> % grade to norm/1
  veh_spd_mps/1 -> Sign/1
  Trigonometric Function2/1 -> Trigonometric Function3/1
  Gravitational Acceleration (m/sec^2)1/1 -> Rolling Resistance Force (N)/2
  % grade to norm/1 -> Trigonometric Function2/1
  Trigonometric Function3/1 -> Rolling Resistance Force (N)/1
  Rolling Resistance Force (N)/1 -> " roll_res_force_N"/1
  Crr/1 -> Rolling Resistance Force (N)/5
  Static Vehicle Mass (kg)/1 -> Rolling Resistance Force (N)/3
  Sign/1 -> Rolling Resistance Force (N)/4
